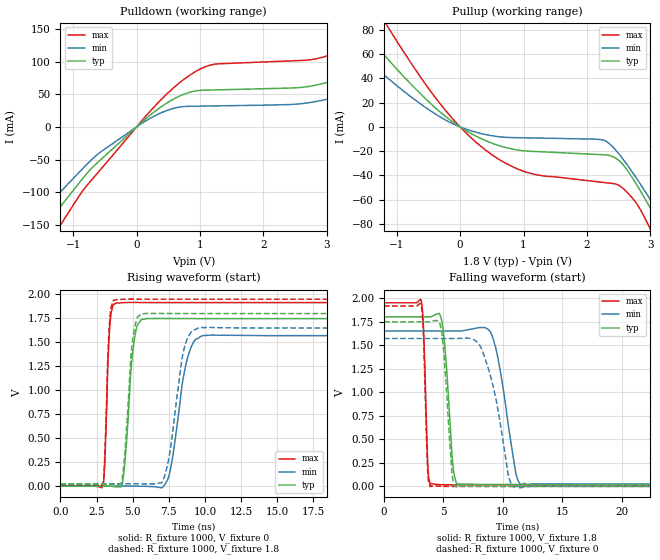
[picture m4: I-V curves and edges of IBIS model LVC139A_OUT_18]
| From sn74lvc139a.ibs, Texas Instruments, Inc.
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[Model]   LVC139A_OUT_18
Model_type  Output
Vref =   0
Rref =   1000
Cref =   30p
Vmeas =   0.9
| variable   typ   min   max
C_comp   6.04pF   2.88pF   12.44pF
| C_pullup   4.75pF   3.40pF   5.59pF
| C_pulldown   7.32pF   2.88pF   12.44pF
[Temperature Range]   40   100   -40
| Ambient temperature   25   85   -40
[Voltage range]   1.8   1.65   1.95
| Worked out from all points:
|   slope of the pulldown table from 0 to 0.27 V, typ, clamps not added: 12.1 ohm
|   slope of the pullup table from 0 to 0.27 V, typ, clamps not added: 33.3 ohm
|   rising waveform, R_fixture 1000, V_fixture 0: 20-80 % time 488ps typ, 888ps min, 260ps max; typ from 0 V to 1.75 V
|   falling waveform, R_fixture 1000, V_fixture 1.8: 20-80 % time 553ps typ, 1.18ns min, 276ps max; typ from 1.8 V to 0.02 V
|   rising waveform, R_fixture 1000, V_fixture 1.8: 20-80 % time 464ps typ, 841ps min, 252ps max; typ from 0.02 V to 1.8 V
|   falling waveform, R_fixture 1000, V_fixture 0: 20-80 % time 551ps typ, 1.45ns min, 267ps max; typ from 1.75 V to 0 V
[Pulldown]
| LVC139A_OUT_18
|   Voltage   I(typ)   I(min)   I(max)
-5.5V     -597.7mA   -511.5mA   -720.2mA
-1.92V    -208.1mA   -170.9mA   -256.6mA
-1.46V    -153.7mA   -125.8mA   -189.4mA
-1.24V    -126.9mA   -103.6mA   -156.4mA
-620mV    -54.96mA   -42.36mA   -71.2mA
55mV      4.891mA    3.664mA    6.376mA
890mV     54.39mA    31.65mA    82.55mA
2.905V    65.74mA    40.4mA     106.1mA
3.915V    104.9mA    72.08mA    156.8mA
4.755V    153.1mA    110.8mA    222.3mA
5.66V     214.2mA    160.5mA    304.8mA
11V       668.1mA    541.1mA    903.2mA
[Pullup]
| LVC139A_OUT_18
|   Voltage   I(typ)   I(min)   I(max)
-5.5V     388.1mA    306.3mA    540.5mA
-2.04V    114mA      85mA       164.6mA
-1.63V    86.5mA     63.62mA    126mA
-1.125V   55.12mA    39.64mA    81.38mA
-295mV    11.44mA    7.609mA    17.81mA
405mV     -11.37mA   -6.347mA   -19.27mA
1.09V     -20.08mA   -9.056mA   -38.07mA
2.265V    -23.01mA   -10.95mA   -45.86mA
2.58V     -31.9mA    -27.46mA   -51.29mA
2.98V     -65.32mA   -58.49mA   -82.31mA
3.295V    -95.62mA   -85.36mA   -117.7mA
11V       -944.3mA   -825.3mA   -1.129A
[Ramp]
| LVC139A_OUT_18
| variable   typ   min   max
dV/dt_r   1.06/5.31E-10   0.96/1.00E-09   1.16/2.81E-10
dV/dt_f   1.09/5.77E-10   1.00/1.26E-09   1.18/2.93E-10
R_load = 1000
[Rising Waveform]
| LVC139A_OUT_18
R_fixture =   1000
C_fixture =   0
L_fixture =   0
V_fixture =   0
V_fixture_min = 0
V_fixture_max = 0
|   Time   V(typ)   V(min)   V(max)
0s        22.65pV    2.842nV    1.798nV
2.94ns    223.2uV    350.2nV    8.573mV
3.415ns   -1.388mV   -12.88uV   1.669V
3.835ns   -7.636mV   -2.675uV   1.909V
4.3ns     46.53mV    113.6uV    1.914V
5.66ns    1.742V     -1.331mV   1.916V
7.475ns   1.749V     90.68mV    1.915V
8.725ns   1.748V     1.3V       1.915V
9.85ns    1.748V     1.57V      1.915V
50ns      1.748V     1.57V      1.915V
[Falling Waveform]
| LVC139A_OUT_18
R_fixture =   1000
C_fixture =   0
L_fixture =   0
V_fixture =   1.8
V_fixture_min = 1.65
V_fixture_max = 1.95
|   Time   V(typ)   V(min)   V(max)
0s        1.8V       1.65V      1.95V
3.14ns    1.8V       1.65V      1.966V
3.68ns    1.799V     1.65V      230.5mV
3.89ns    1.801V     1.65V      27.31mV
4.89ns    1.735V     1.65V      17.5mV
5.755ns   275.4mV    1.65V      16.32mV
6.185ns   20.09mV    1.649V     16.37mV
9.05ns    19.99mV    1.611V     16.54mV
11.55ns   19.75mV    18.35mV    16.56mV
50ns      19.81mV    24.07mV    16.56mV
[Rising Waveform]
| LVC139A_OUT_18
R_fixture =   1000
C_fixture =   0
L_fixture =   0
V_fixture =   1.8
V_fixture_min = 1.65
V_fixture_max = 1.95
|   Time   V(typ)   V(min)   V(max)
0s        19.81mV    24.07mV    16.56mV
2.925ns   20mV       24.07mV    25.96mV
3.39ns    18.69mV    24.06mV    1.69V
3.825ns   14.73mV    24.08mV    1.945V
4.265ns   60.93mV    24.16mV    1.949V
5.63ns    1.8V       23.03mV    1.951V
7.15ns    1.801V     81.06mV    1.95V
8.535ns   1.8V       1.422V     1.95V
9.59ns    1.8V       1.653V     1.95V
50ns      1.8V       1.65V      1.95V
[Falling Waveform]
| LVC139A_OUT_18
R_fixture =   1000
C_fixture =   0
L_fixture =   0
V_fixture =   0
V_fixture_min = 0
V_fixture_max = 0
|   Time   V(typ)   V(min)   V(max)
0s        1.748V     1.57V      1.915V
3.12ns    1.748V     1.57V      1.924V
3.675ns   1.747V     1.57V      160.8mV
3.895ns   1.748V     1.57V      -2.364mV
4.86ns    1.632V     1.57V      600.2uV
5.715ns   141.8mV    1.57V      -162.4uV
6.145ns   -7.552mV   1.57V      -160.8uV
8.32ns    181.1uV    1.425V     -26.82uV
10.92ns   -30.36uV   -6.41mV    -142.8nV
50ns      -5.632nV   7.39nV     -223.3pV
